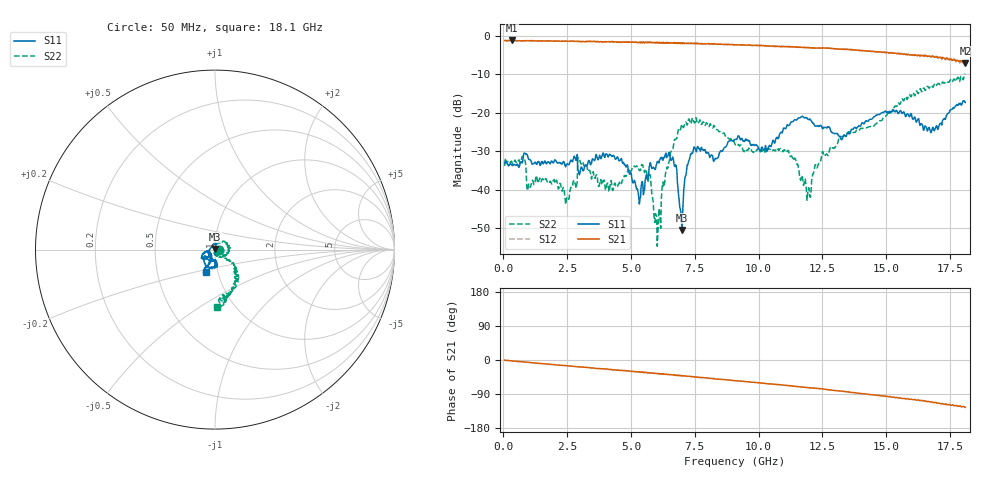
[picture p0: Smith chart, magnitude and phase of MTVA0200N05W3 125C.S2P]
! Network Analyzer HP8720D.06.14 Serial No. US36140669
! 17 Jan 2005  14:11:06
! Frequency  S11  S21  S12  S22
# HZ  S  DB R 50
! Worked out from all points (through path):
!   801 points, 50 MHz to 18.1 GHz, reference 50 ohm
!   highest |S21| = -1.12 dB at 343.3 MHz (marker M1); lowest = -7.0 dB at 18.1 GHz (marker M2)
!   group delay of S21, straight-line fit = 18.3 ps
!   lowest |S11| = -50.5 dB at 6.999 GHz (marker M3), VSWR 1.01, Z = 49.9 + j0.28 ohm
!   |S11| at or under -10 dB: start of sweep to end of sweep
!   |S22| runs from -54.8 to -9.9 dB; largest |S21 - S12| = 0.028
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5e7  -32.99 -10.1  -1.14 -0.6  -1.17 -1.2  -33.85 -4.5
3.433125e8  -33.65 -6.7  -1.12 -2.6  -1.14 -3.0  -33.06 -13.6
2.48675e9  -33.33 -3.4  -1.32 -15.2  -1.31 -15.5  -41.96 23.9
3.073375e9  -34.23 4.4  -1.39 -18.7  -1.37 -18.9  -32.87 -57.6
4.088688e9  -31.28 -17.6  -1.46 -24.1  -1.46 -24.7  -38.32 -57.5
5.2845e9  -40.99 -30.4  -1.67 -31.8  -1.61 -32.0  -34.38 -42.3
5.510125e9  -40.37 -66.1  -1.69 -33.6  -1.71 -33.6  -34.89 -54.4
6.074188e9  -32.74 -93.4  -1.79 -36.8  -1.77 -36.9  -48.57 41.4
6.683375e9  -33.26 -92.6  -1.66 -39.2  -1.67 -39.4  -27.67 65.4
6.99925e9  -50.53 109.3  -1.80 -42.4  -1.85 -42.7  -22.97 37.5
7.17975e9  -34.83 83.7  -1.88 -42.2  -1.85 -42.6  -22.88 22.4
7.427938e9  -30.20 82.2  -1.97 -44.3  -1.94 -44.7  -21.70 5.3
8.307875e9  -31.81 152.2  -2.05 -50.0  -2.00 -50.3  -24.17 -36.5
9.075e9  -26.93 -139.8  -2.26 -54.3  -2.26 -54.8  -28.14 -67.2
1.027081e10  -28.53 -146.8  -2.49 -62.1  -2.49 -62.2  -29.71 -57.2
1.108306e10  -23.84 -160.5  -2.71 -66.8  -2.74 -67.3  -30.34 -58.4
1.1963e10  -21.73 -144.0  -2.96 -73.5  -3.01 -73.6  -39.54 -6.1
1.209838e10  -22.49 -136.6  -3.03 -74.1  -3.05 -74.3  -36.74 -5.7
1.32265e10  -26.86 -115.5  -3.38 -82.0  -3.38 -82.4  -26.16 -14.4
1.509919e10  -19.89 -112.1  -4.41 -97.0  -4.26 -97.6  -20.46 -39.1
1.681394e10  -23.83 -100.5  -5.22 -111.2  -5.06 -111.9  -13.30 -61.3
1.81e10  -17.28 -112.7  -7.00 -125.0  -6.70 -125.1  -9.95 -88.2
